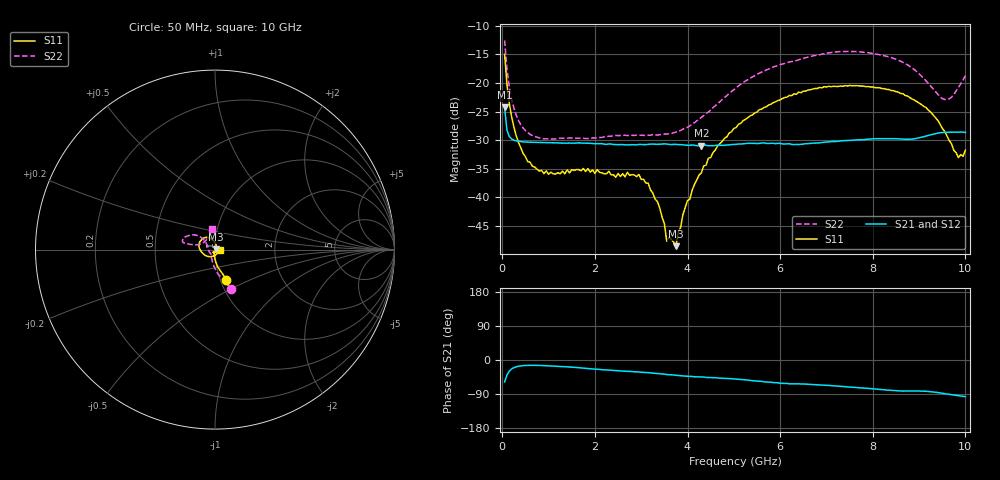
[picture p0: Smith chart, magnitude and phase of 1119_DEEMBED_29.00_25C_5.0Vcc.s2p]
!Hittite Microwave Corp.
!Digital Attenuator/PhaseShifter Rev 1.4.0
!Filename: C:\DATA\DATA\1119_DEEMBED_29.00_25C_5.0Vcc.s2p
!VNA ID: Agilent Technologies,N5224A,MY51441122,A.10.45.03
!Device type:
!2 Port Calibration.
!Temp(C): 25
!Lot Number:
!Serial Number:
!Operator:
!Misc:
!Attenuator:  29.000
# GHZ S DB R 50.0
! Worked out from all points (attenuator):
!   200 points, 50 MHz to 10 GHz, reference 50 ohm
!   highest |S21| = -24.22 dB at 50 MHz (marker M1); lowest = -31.0 dB at 4.3 GHz (marker M2)
!   lowest |S11| = -48.5 dB at 3.75 GHz (marker M3), VSWR 1.01, Z = 50.4 + j0.129 ohm
!   |S11| at or under -10 dB: start of sweep to end of sweep
!   |S22| runs from -29.8 to -12.6 dB; largest |S21 - S12| = 0.00011
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0.05  -14.96 -69.0  -24.22 -58.0  -24.22 -58.0  -12.55 -67.5
0.1  -20.21 -81.0  -28.22 -40.1  -28.20 -40.0  -17.51 -84.0
0.2  -25.86 -90.7  -29.79 -23.8  -29.78 -23.9  -22.78 -100.6
0.35  -30.41 -98.2  -30.20 -16.5  -30.20 -16.5  -26.57 -114.7
0.55  -33.75 -106.9  -30.34 -14.2  -30.33 -14.1  -28.66 -126.5
1  -35.97 -117.1  -30.43 -15.3  -30.45 -15.3  -29.74 -137.3
1.75  -34.96 -121.5  -30.52 -21.5  -30.53 -21.5  -29.67 -140.9
2.95  -36.00 -97.0  -30.74 -31.5  -30.75 -31.6  -29.14 -160.2
3.15  -37.51 -89.3  -30.73 -33.3  -30.74 -33.4  -29.13 -166.2
3.4  -41.88 -84.1  -30.70 -36.1  -30.70 -36.2  -29.05 -173.8
3.5  -44.62 -71.6  -30.64 -37.3  -30.65 -37.3  -28.94 -177.3
3.55  -47.66 -54.4  -30.68 -38.4  -30.69 -38.5  -28.93 -179.2
3.75  -48.55 20.0  -30.74 -40.3  -30.74 -40.4  -28.58 173.0
4  -40.55 49.4  -30.89 -42.8  -30.89 -42.8  -27.76 161.8
4.3  -35.71 67.7  -30.99 -44.6  -30.99 -44.7  -25.99 150.4
5.05  -27.79 91.5  -30.73 -50.3  -30.74 -50.4  -20.83 138.6
6.7  -21.07 132.4  -30.52 -64.7  -30.53 -64.7  -15.26 153.8
8.35  -21.14 174.6  -29.75 -79.6  -29.75 -79.6  -15.44 168.1
9.15  -24.29 -145.8  -29.28 -82.5  -29.29 -82.6  -19.62 165.4
9.55  -28.43 -105.2  -28.63 -88.9  -28.65 -89.0  -22.87 138.1
9.85  -33.05 -41.2  -28.59 -94.0  -28.59 -94.0  -20.77 105.8
10  -31.77 0.7  -28.64 -96.7  -28.64 -96.7  -18.74 98.2
